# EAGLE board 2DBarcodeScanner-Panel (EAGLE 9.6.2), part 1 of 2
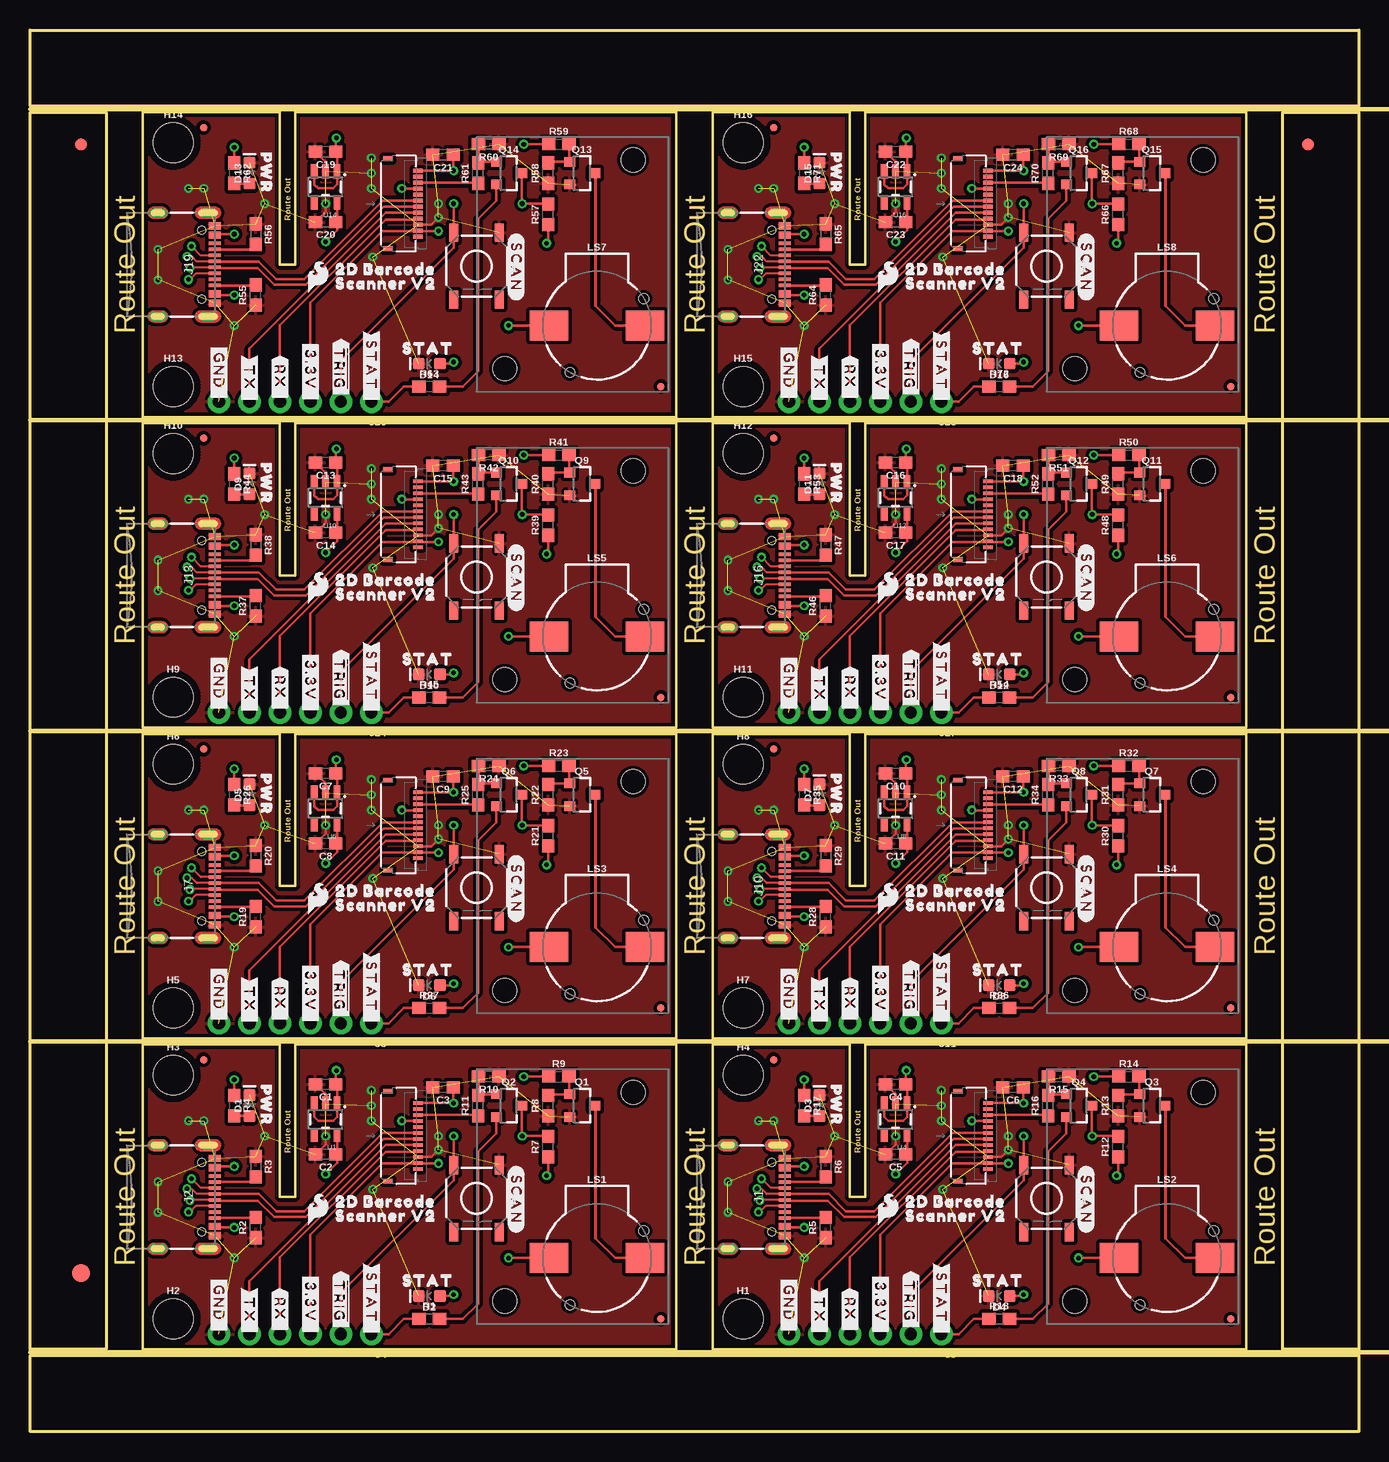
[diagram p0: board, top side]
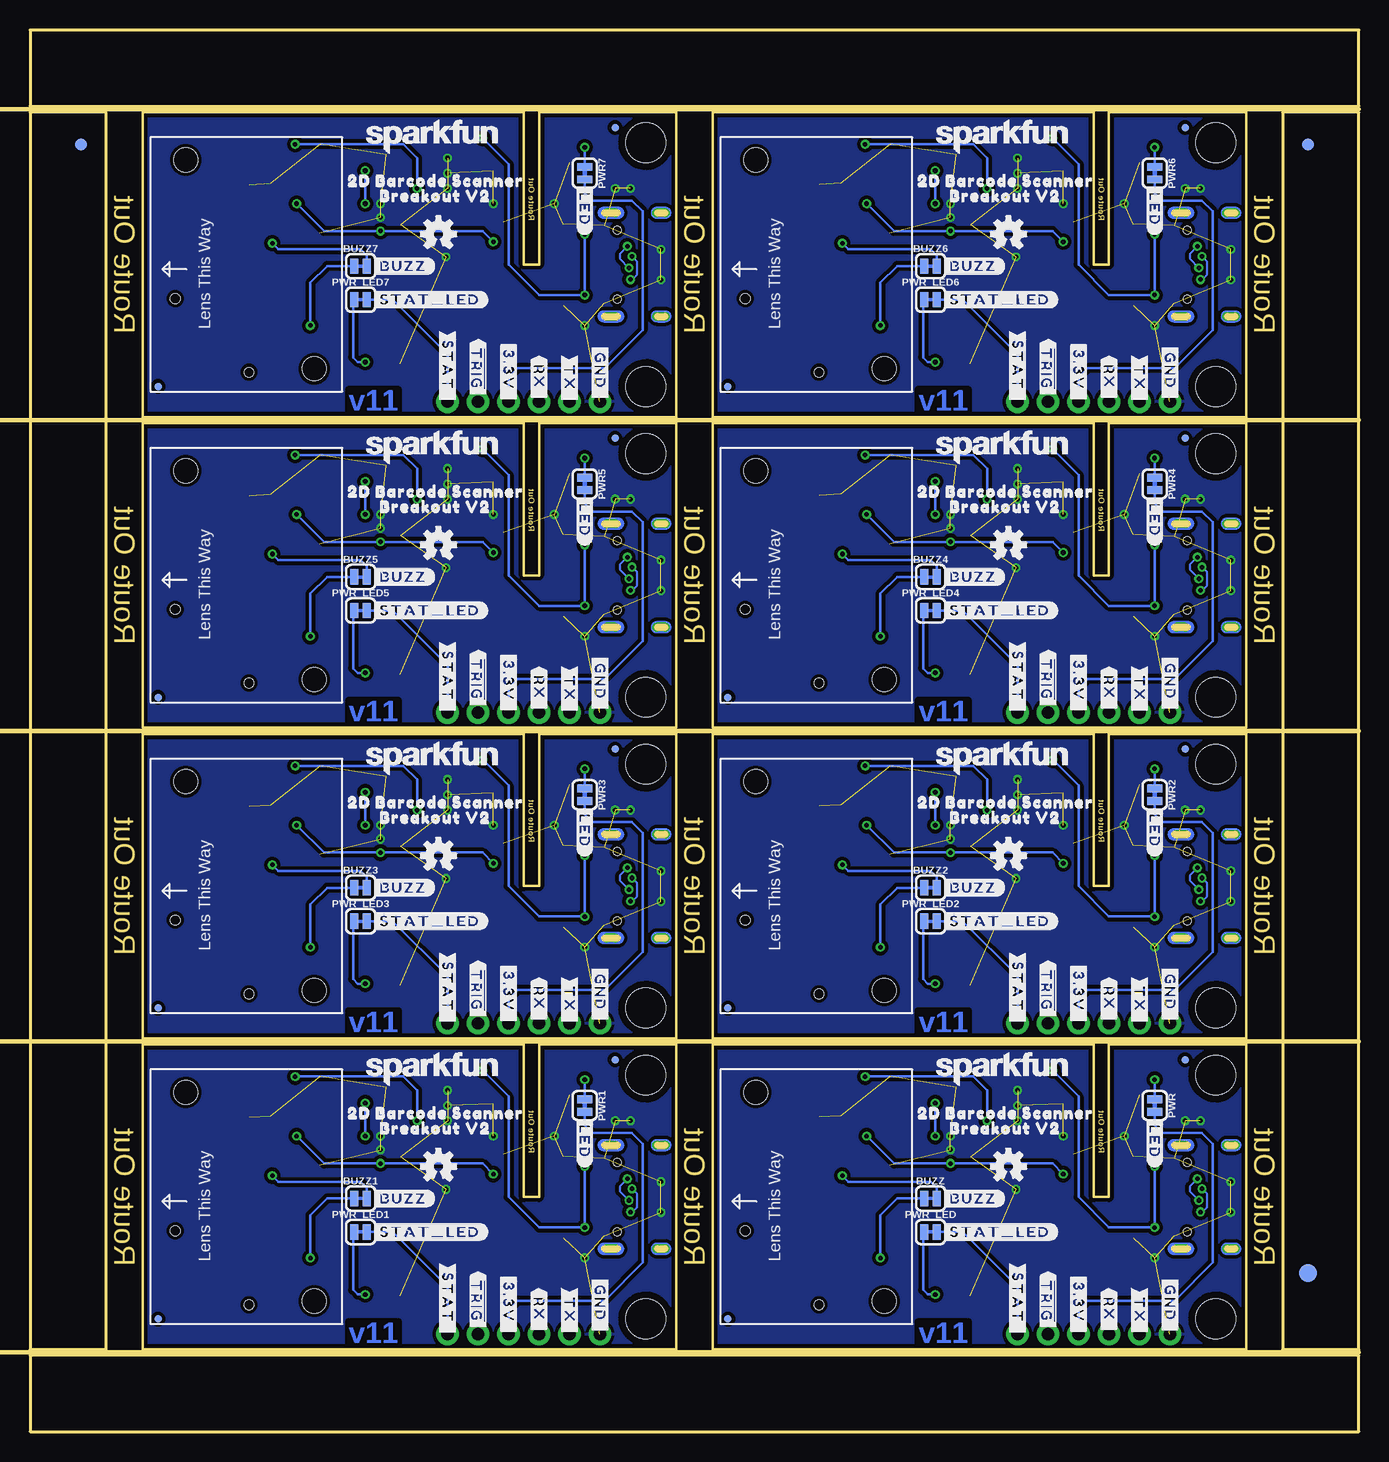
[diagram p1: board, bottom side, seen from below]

Size 110.74 x 116.84 mm. Coordinates in mm from the lower left corner, seen from the top.
Outline: 80 segments
Copper layers (1*16): Top 0.035mm / dielectric 1.5mm / Bottom 0.035mm
Design rules "2DBarcodeScanner": minimum track width 7mil, minimum drill 0.3mm, track to track 7mil, track to pad 7mil, pad to pad 7mil, via to via 7mil, smd to smd 7mil, copper to edge 7mil, drill to drill 7mil, minimum pad ring 7mil, minimum via ring 7mil, stop-mask expansion 3mil, vias tented up to drill 25mil, thermal gap 10mil
Net classes: 1 power: width 0.178 mm
Milling: 5 lines

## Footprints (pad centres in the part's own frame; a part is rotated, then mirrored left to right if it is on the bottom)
SMT-JUMPER_2_NC_TRACE_SILK = smd 0.66 x 1.27: 1 -0.521,0; 2 0.521,0
0603 = smd 1.1 x 1: 1 -0.85,0; 2 0.85,0
LED-0603 = smd 1 x 1: A -0.877,0; C 0.877,0
FIDUCIAL-1X2 = smd 1 x 1: 1 0,0
FIDUCIAL-1.5X3 = smd 1.5 x 1.5: 1 0,0
FIDUCIAL-MICRO = smd 0.635 x 0.635: 1 0,0
STAND-OFF = hole 3.302: 0,0
USB-C-16P-2LAYER-PADS = smd 0.3 x 1: A5 -1.25,-0.34; A6 -0.25,-0.34; A7 0.25,-0.34; A8 1.25,-0.34; B5 1.75,-0.34; B6 0.75,-0.34; B7 -0.75,-0.34; B8 -1.75,-0.34 | smd 0.6 x 1: GND -3.225,-0.34; GND2 3.225,-0.34; VBUS1 -2.45,-0.34; VBUS2 2.45,-0.34 | drill 0.4 pad 0.6 long: SHLD1 -4.318,-0.915; SHLD2 4.318,-0.915; SHLD3 -4.318,-5.095; SHLD4 4.318,-5.095 | hole 0.65: -2.89,-1.445; 2.89,-1.445
FPC_12_0.5MM = smd 0.3 x 0.8: 1 -2.75,1.35; 2 -2.25,1.35; 3 -1.75,1.35; 4 -1.25,1.35; 5 -0.75,1.35; 6 -0.25,1.35; 7 0.25,1.35; 8 0.75,1.35; 9 1.25,1.35; 10 1.75,1.35; 11 2.25,1.35; 12 2.75,1.35 | smd 0.4 x 0.8: MP1 -3.75,-1.15; MP2 3.75,-1.15
1X06_NO_SILK = drill 1.016 pad 1.88: 1 0,0; 2 2.54,0; 3 5.08,0; 4 7.62,0; 5 10.16,0; 6 12.7,0
BUZZER-CCV = smd 3.2 x 2.5: + 4,0; - -4,0 | hole 0.8: -3.9,-2.25; 2.25,3.9
SOT23-3 = smd 0.8 x 0.9: 1 -0.95,-1; 2 0.95,-1; 3 0,1.1
TACTILE_SWITCH_SMD_5.2MM = smd 1.524 x 0.762: 1 -2.794,1.905; 2 2.794,1.905; 3 -2.794,-1.905; 4 2.794,-1.905
SOT23-5 = smd 0.55 x 1.2: 1 -0.95,-1.3; 2 0,-1.3; 3 0.95,-1.3; 4 0.95,1.3; 5 -0.95,1.3
BARCODE_SCANNER_MOUNT = hole 2: -5.65,8.3; 5.05,-9.1

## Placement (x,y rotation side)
BUZZ  JUMPER-SMT_2_NC_TRACE_SILK  [SMT-JUMPER_2_NC_TRACE_SILK]  35.69,19.43 0 bottom
BUZZ1  JUMPER-SMT_2_NC_TRACE_SILK  [SMT-JUMPER_2_NC_TRACE_SILK]  83.19,19.43 0 bottom
BUZZ2  JUMPER-SMT_2_NC_TRACE_SILK  [SMT-JUMPER_2_NC_TRACE_SILK]  35.69,45.34 0 bottom
BUZZ3  JUMPER-SMT_2_NC_TRACE_SILK  [SMT-JUMPER_2_NC_TRACE_SILK]  83.19,45.34 0 bottom
BUZZ4  JUMPER-SMT_2_NC_TRACE_SILK  [SMT-JUMPER_2_NC_TRACE_SILK]  35.69,71.25 0 bottom
BUZZ5  JUMPER-SMT_2_NC_TRACE_SILK  [SMT-JUMPER_2_NC_TRACE_SILK]  83.19,71.25 0 bottom
BUZZ6  JUMPER-SMT_2_NC_TRACE_SILK  [SMT-JUMPER_2_NC_TRACE_SILK]  35.69,97.16 0 bottom
BUZZ7  JUMPER-SMT_2_NC_TRACE_SILK  [SMT-JUMPER_2_NC_TRACE_SILK]  83.19,97.16 0 bottom
C1  1.0uF  [0603]  24.64,28.96 180 top
C2  1.0uF  [0603]  24.64,23.11 180 top
C3  0.1uF  [0603]  34.42,28.7 180 top
C4  1.0uF  [0603]  72.14,28.96 180 top
C5  1.0uF  [0603]  72.14,23.11 180 top
C6  0.1uF  [0603]  81.91,28.7 180 top
C7  1.0uF  [0603]  24.64,54.86 180 top
C8  1.0uF  [0603]  24.64,49.02 180 top
C9  0.1uF  [0603]  34.42,54.61 180 top
C10  1.0uF  [0603]  72.14,54.86 180 top
C11  1.0uF  [0603]  72.14,49.02 180 top
C12  0.1uF  [0603]  81.91,54.61 180 top
C13  1.0uF  [0603]  24.64,80.77 180 top
C14  1.0uF  [0603]  24.64,74.93 180 top
C15  0.1uF  [0603]  34.42,80.52 180 top
C16  1.0uF  [0603]  72.14,80.77 180 top
C17  1.0uF  [0603]  72.14,74.93 180 top
C18  0.1uF  [0603]  81.91,80.52 180 top
C19  1.0uF  [0603]  24.64,106.68 180 top
C20  1.0uF  [0603]  24.64,100.84 180 top
C21  0.1uF  [0603]  34.42,106.43 180 top
C22  1.0uF  [0603]  72.14,106.68 180 top
C23  1.0uF  [0603]  72.14,100.84 180 top
C24  0.1uF  [0603]  81.91,106.43 180 top
D1  RED  [LED-0603]  18.29,27.18 90 top
D2  GREEN  [LED-0603]  33.27,11.3 180 top
D3  RED  [LED-0603]  65.79,27.18 90 top
D4  GREEN  [LED-0603]  80.77,11.3 180 top
D5  RED  [LED-0603]  18.29,53.09 90 top
D6  GREEN  [LED-0603]  33.27,37.21 180 top
D7  RED  [LED-0603]  65.79,53.09 90 top
D8  GREEN  [LED-0603]  80.77,37.21 180 top
D9  RED  [LED-0603]  18.29,78.99 90 top
D10  GREEN  [LED-0603]  33.27,63.12 180 top
D11  RED  [LED-0603]  65.79,78.99 90 top
D12  GREEN  [LED-0603]  80.77,63.12 180 top
D13  RED  [LED-0603]  18.29,104.9 90 top
D14  GREEN  [LED-0603]  33.27,89.03 180 top
D15  RED  [LED-0603]  65.79,104.9 90 top
D16  GREEN  [LED-0603]  80.77,89.03 180 top
E$1  [FIDUCIAL-1X2]  4.23,107.31 0 top
E$2  [FIDUCIAL-1X2]  4.23,107.31 0 bottom
E$3  [FIDUCIAL-1X2]  106.51,107.31 0 top
E$4  [FIDUCIAL-1X2]  106.51,107.31 0 bottom
E$5  [FIDUCIAL-1.5X3]  4.23,13.21 0 top
E$6  [FIDUCIAL-1.5X3]  4.23,13.21 0 bottom
FD1  FIDUCIALUFIDUCIAL  [FIDUCIAL-MICRO]  14.48,30.99 0 top
FD2  FIDUCIALUFIDUCIAL  [FIDUCIAL-MICRO]  52.58,9.4 0 top
FD3  FIDUCIALUFIDUCIAL  [FIDUCIAL-MICRO]  52.58,9.4 0 bottom
FD4  FIDUCIALUFIDUCIAL  [FIDUCIAL-MICRO]  14.48,30.99 0 bottom
FD5  FIDUCIALUFIDUCIAL  [FIDUCIAL-MICRO]  61.98,30.99 0 top
FD6  FIDUCIALUFIDUCIAL  [FIDUCIAL-MICRO]  100.08,9.4 0 top
FD7  FIDUCIALUFIDUCIAL  [FIDUCIAL-MICRO]  100.08,9.4 0 bottom
FD8  FIDUCIALUFIDUCIAL  [FIDUCIAL-MICRO]  61.98,30.99 0 bottom
FD9  FIDUCIALUFIDUCIAL  [FIDUCIAL-MICRO]  14.48,56.9 0 top
FD10  FIDUCIALUFIDUCIAL  [FIDUCIAL-MICRO]  52.58,35.31 0 top
FD11  FIDUCIALUFIDUCIAL  [FIDUCIAL-MICRO]  52.58,35.31 0 bottom
FD12  FIDUCIALUFIDUCIAL  [FIDUCIAL-MICRO]  14.48,56.9 0 bottom
FD13  FIDUCIALUFIDUCIAL  [FIDUCIAL-MICRO]  61.98,56.9 0 top
FD14  FIDUCIALUFIDUCIAL  [FIDUCIAL-MICRO]  100.08,35.31 0 top
FD15  FIDUCIALUFIDUCIAL  [FIDUCIAL-MICRO]  100.08,35.31 0 bottom
FD16  FIDUCIALUFIDUCIAL  [FIDUCIAL-MICRO]  61.98,56.9 0 bottom
FD17  FIDUCIALUFIDUCIAL  [FIDUCIAL-MICRO]  14.48,82.8 0 top
FD18  FIDUCIALUFIDUCIAL  [FIDUCIAL-MICRO]  52.58,61.21 0 top
FD19  FIDUCIALUFIDUCIAL  [FIDUCIAL-MICRO]  52.58,61.21 0 bottom
FD20  FIDUCIALUFIDUCIAL  [FIDUCIAL-MICRO]  14.48,82.8 0 bottom
FD21  FIDUCIALUFIDUCIAL  [FIDUCIAL-MICRO]  61.98,82.8 0 top
FD22  FIDUCIALUFIDUCIAL  [FIDUCIAL-MICRO]  100.08,61.21 0 top
FD23  FIDUCIALUFIDUCIAL  [FIDUCIAL-MICRO]  100.08,61.21 0 bottom
FD24  FIDUCIALUFIDUCIAL  [FIDUCIAL-MICRO]  61.98,82.8 0 bottom
FD25  FIDUCIALUFIDUCIAL  [FIDUCIAL-MICRO]  14.48,108.71 0 top
FD26  FIDUCIALUFIDUCIAL  [FIDUCIAL-MICRO]  52.58,87.12 0 top
FD27  FIDUCIALUFIDUCIAL  [FIDUCIAL-MICRO]  52.58,87.12 0 bottom
FD28  FIDUCIALUFIDUCIAL  [FIDUCIAL-MICRO]  14.48,108.71 0 bottom
FD29  FIDUCIALUFIDUCIAL  [FIDUCIAL-MICRO]  61.98,108.71 0 top
FD30  FIDUCIALUFIDUCIAL  [FIDUCIAL-MICRO]  100.08,87.12 0 top
FD31  FIDUCIALUFIDUCIAL  [FIDUCIAL-MICRO]  100.08,87.12 0 bottom
FD32  FIDUCIALUFIDUCIAL  [FIDUCIAL-MICRO]  61.98,108.71 0 bottom
H1  STAND-OFF  [STAND-OFF]  59.44,9.4 0 top
H2  STAND-OFF  [STAND-OFF]  11.94,9.4 0 top
H3  STAND-OFF  [STAND-OFF]  11.94,29.72 0 top
H4  STAND-OFF  [STAND-OFF]  59.44,29.72 0 top
H5  STAND-OFF  [STAND-OFF]  11.94,35.31 0 top
H6  STAND-OFF  [STAND-OFF]  11.94,55.63 0 top
H7  STAND-OFF  [STAND-OFF]  59.44,35.31 0 top
H8  STAND-OFF  [STAND-OFF]  59.44,55.63 0 top
H9  STAND-OFF  [STAND-OFF]  11.94,61.21 0 top
H10  STAND-OFF  [STAND-OFF]  11.94,81.53 0 top
H11  STAND-OFF  [STAND-OFF]  59.44,61.21 0 top
H12  STAND-OFF  [STAND-OFF]  59.44,81.53 0 top
H13  STAND-OFF  [STAND-OFF]  11.94,87.12 0 top
H14  STAND-OFF  [STAND-OFF]  11.94,107.44 0 top
H15  STAND-OFF  [STAND-OFF]  59.44,87.12 0 top
H16  STAND-OFF  [STAND-OFF]  59.44,107.44 0 top
J1  [USB-C-16P-2LAYER-PADS]  63.25,19.56 270 top
J2  [USB-C-16P-2LAYER-PADS]  15.75,19.56 270 top
J3  [FPC_12_0.5MM]  30.99,24.64 270 top
J4  [1X06_NO_SILK]  28.45,8.13 180 top
J5  [1X06_NO_SILK]  75.95,8.13 180 top
J6  [FPC_12_0.5MM]  78.49,24.64 270 top
J7  [USB-C-16P-2LAYER-PADS]  15.75,45.47 270 top
J8  [1X06_NO_SILK]  28.45,34.04 180 top
J9  [FPC_12_0.5MM]  30.99,50.55 270 top
J10  [USB-C-16P-2LAYER-PADS]  63.25,45.47 270 top
J11  [1X06_NO_SILK]  75.95,34.04 180 top
J12  [FPC_12_0.5MM]  78.49,50.55 270 top
J13  [USB-C-16P-2LAYER-PADS]  15.75,71.37 270 top
J14  [1X06_NO_SILK]  28.45,59.94 180 top
J15  [FPC_12_0.5MM]  30.99,76.45 270 top
J16  [USB-C-16P-2LAYER-PADS]  63.25,71.37 270 top
J17  [1X06_NO_SILK]  75.95,59.94 180 top
J18  [FPC_12_0.5MM]  78.49,76.45 270 top
J19  [USB-C-16P-2LAYER-PADS]  15.75,97.28 270 top
J20  [1X06_NO_SILK]  28.45,85.85 180 top
J21  [FPC_12_0.5MM]  30.99,102.36 270 top
J22  [USB-C-16P-2LAYER-PADS]  63.25,97.28 270 top
J23  [1X06_NO_SILK]  75.95,85.85 180 top
J24  [FPC_12_0.5MM]  78.49,102.36 270 top
LOGO1  OSHW-LOGOS  [OSHW-LOGO-S]  29.21,22.1 0 bottom
LOGO2  SFE_LOGO_FLAME.1_INCH  [SFE_LOGO_FLAME_.1]  24,18.54 0 top
LOGO3  SFE_LOGO_NAME.1_INCH  [SFE_LOGO_NAME_.1]  29.72,30.23 0 bottom
LOGO4  OSHW-LOGOS  [OSHW-LOGO-S]  76.71,22.1 0 bottom
LOGO5  SFE_LOGO_FLAME.1_INCH  [SFE_LOGO_FLAME_.1]  71.5,18.54 0 top
LOGO6  SFE_LOGO_NAME.1_INCH  [SFE_LOGO_NAME_.1]  77.22,30.23 0 bottom
LOGO7  OSHW-LOGOS  [OSHW-LOGO-S]  29.21,48.01 0 bottom
LOGO8  SFE_LOGO_FLAME.1_INCH  [SFE_LOGO_FLAME_.1]  24,44.45 0 top
LOGO9  SFE_LOGO_NAME.1_INCH  [SFE_LOGO_NAME_.1]  29.72,56.13 0 bottom
LOGO10  OSHW-LOGOS  [OSHW-LOGO-S]  76.71,48.01 0 bottom
LOGO11  SFE_LOGO_FLAME.1_INCH  [SFE_LOGO_FLAME_.1]  71.5,44.45 0 top
LOGO12  SFE_LOGO_NAME.1_INCH  [SFE_LOGO_NAME_.1]  77.22,56.13 0 bottom
LOGO13  OSHW-LOGOS  [OSHW-LOGO-S]  29.21,73.91 0 bottom
LOGO14  SFE_LOGO_FLAME.1_INCH  [SFE_LOGO_FLAME_.1]  24,70.36 0 top
LOGO15  SFE_LOGO_NAME.1_INCH  [SFE_LOGO_NAME_.1]  29.72,82.04 0 bottom
LOGO16  OSHW-LOGOS  [OSHW-LOGO-S]  76.71,73.91 0 bottom
LOGO17  SFE_LOGO_FLAME.1_INCH  [SFE_LOGO_FLAME_.1]  71.5,70.36 0 top
LOGO18  SFE_LOGO_NAME.1_INCH  [SFE_LOGO_NAME_.1]  77.22,82.04 0 bottom
LOGO19  OSHW-LOGOS  [OSHW-LOGO-S]  29.21,99.82 0 bottom
LOGO20  SFE_LOGO_FLAME.1_INCH  [SFE_LOGO_FLAME_.1]  24,96.27 0 top
LOGO21  SFE_LOGO_NAME.1_INCH  [SFE_LOGO_NAME_.1]  29.72,107.95 0 bottom
LOGO22  OSHW-LOGOS  [OSHW-LOGO-S]  76.71,99.82 0 bottom
LOGO23  SFE_LOGO_FLAME.1_INCH  [SFE_LOGO_FLAME_.1]  71.5,96.27 0 top
LOGO24  SFE_LOGO_NAME.1_INCH  [SFE_LOGO_NAME_.1]  77.22,107.95 0 bottom
LS1  BUZZER-SMD  [BUZZER-CCV]  47.24,14.48 180 top
LS2  BUZZER-SMD  [BUZZER-CCV]  94.74,14.48 180 top
LS3  BUZZER-SMD  [BUZZER-CCV]  47.24,40.39 180 top
LS4  BUZZER-SMD  [BUZZER-CCV]  94.74,40.39 180 top
LS5  BUZZER-SMD  [BUZZER-CCV]  47.24,66.29 180 top
LS6  BUZZER-SMD  [BUZZER-CCV]  94.74,66.29 180 top
LS7  BUZZER-SMD  [BUZZER-CCV]  47.24,92.2 180 top
LS8  BUZZER-SMD  [BUZZER-CCV]  94.74,92.2 180 top
PWR  JUMPER-SMT_2_NC_TRACE_SILK  [SMT-JUMPER_2_NC_TRACE_SILK]  17.02,27.18 270 bottom
PWR1  JUMPER-SMT_2_NC_TRACE_SILK  [SMT-JUMPER_2_NC_TRACE_SILK]  64.52,27.18 270 bottom
PWR2  JUMPER-SMT_2_NC_TRACE_SILK  [SMT-JUMPER_2_NC_TRACE_SILK]  17.02,53.09 270 bottom
PWR3  JUMPER-SMT_2_NC_TRACE_SILK  [SMT-JUMPER_2_NC_TRACE_SILK]  64.52,53.09 270 bottom
PWR4  JUMPER-SMT_2_NC_TRACE_SILK  [SMT-JUMPER_2_NC_TRACE_SILK]  17.02,78.99 270 bottom
PWR5  JUMPER-SMT_2_NC_TRACE_SILK  [SMT-JUMPER_2_NC_TRACE_SILK]  64.52,78.99 270 bottom
PWR6  JUMPER-SMT_2_NC_TRACE_SILK  [SMT-JUMPER_2_NC_TRACE_SILK]  17.02,104.9 270 bottom
PWR7  JUMPER-SMT_2_NC_TRACE_SILK  [SMT-JUMPER_2_NC_TRACE_SILK]  64.52,104.9 270 bottom
PWR_LED  JUMPER-SMT_2_NC_TRACE_SILK  [SMT-JUMPER_2_NC_TRACE_SILK]  35.69,16.64 0 bottom
PWR_LED1  JUMPER-SMT_2_NC_TRACE_SILK  [SMT-JUMPER_2_NC_TRACE_SILK]  83.19,16.64 0 bottom
PWR_LED2  JUMPER-SMT_2_NC_TRACE_SILK  [SMT-JUMPER_2_NC_TRACE_SILK]  35.69,42.54 0 bottom
PWR_LED3  JUMPER-SMT_2_NC_TRACE_SILK  [SMT-JUMPER_2_NC_TRACE_SILK]  83.19,42.54 0 bottom
PWR_LED4  JUMPER-SMT_2_NC_TRACE_SILK  [SMT-JUMPER_2_NC_TRACE_SILK]  35.69,68.45 0 bottom
PWR_LED5  JUMPER-SMT_2_NC_TRACE_SILK  [SMT-JUMPER_2_NC_TRACE_SILK]  83.19,68.45 0 bottom
PWR_LED6  JUMPER-SMT_2_NC_TRACE_SILK  [SMT-JUMPER_2_NC_TRACE_SILK]  35.69,94.36 0 bottom
PWR_LED7  JUMPER-SMT_2_NC_TRACE_SILK  [SMT-JUMPER_2_NC_TRACE_SILK]  83.19,94.36 0 bottom
Q1  600mA/40V  [SOT23-3]  45.97,27.18 270 top
Q2  600mA/40V  [SOT23-3]  39.88,27.18 270 top
Q3  600mA/40V  [SOT23-3]  93.47,27.18 270 top
Q4  600mA/40V  [SOT23-3]  87.38,27.18 270 top
Q5  600mA/40V  [SOT23-3]  45.97,53.09 270 top
Q6  600mA/40V  [SOT23-3]  39.88,53.09 270 top
Q7  600mA/40V  [SOT23-3]  93.47,53.09 270 top
Q8  600mA/40V  [SOT23-3]  87.38,53.09 270 top
Q9  600mA/40V  [SOT23-3]  45.97,78.99 270 top
Q10  600mA/40V  [SOT23-3]  39.88,78.99 270 top
Q11  600mA/40V  [SOT23-3]  93.47,78.99 270 top
Q12  600mA/40V  [SOT23-3]  87.38,78.99 270 top
Q13  600mA/40V  [SOT23-3]  45.97,104.9 270 top
Q14  600mA/40V  [SOT23-3]  39.88,104.9 270 top
Q15  600mA/40V  [SOT23-3]  93.47,104.9 270 top
Q16  600mA/40V  [SOT23-3]  87.38,104.9 270 top
R1  100  [0603]  33.27,9.4 0 top
R2  5.1k  [0603]  18.8,17.02 90 top
R3  5.1k  [0603]  18.8,22.1 270 top
R4  1k  [0603]  17.02,27.18 270 top
R5  5.1k  [0603]  66.29,17.02 90 top
R6  5.1k  [0603]  66.29,22.1 270 top
R7  10  [0603]  43.18,23.75 90 top
R8  10k  [0603]  43.18,27.18 90 top
R9  1k  [0603]  44.07,29.59 0 top
R10  10k  [0603]  38.23,29.59 180 top
R11  1k  [0603]  37.34,27.18 90 top
R12  10  [0603]  90.68,23.75 90 top
R13  10k  [0603]  90.68,27.18 90 top
R14  1k  [0603]  91.57,29.59 0 top
R15  10k  [0603]  85.72,29.59 180 top
R16  1k  [0603]  84.84,27.18 90 top
R17  1k  [0603]  64.52,27.18 270 top
R18  100  [0603]  80.77,9.4 0 top
R19  5.1k  [0603]  18.8,42.93 90 top
R20  5.1k  [0603]  18.8,48.01 270 top
R21  10  [0603]  43.18,49.66 90 top
R22  10k  [0603]  43.18,53.09 90 top
R23  1k  [0603]  44.07,55.5 0 top
R24  10k  [0603]  38.23,55.5 180 top
R25  1k  [0603]  37.34,53.09 90 top
R26  1k  [0603]  17.02,53.09 270 top
R27  100  [0603]  33.27,35.31 0 top
R28  5.1k  [0603]  66.29,42.93 90 top
R29  5.1k  [0603]  66.29,48.01 270 top
R30  10  [0603]  90.68,49.66 90 top
R31  10k  [0603]  90.68,53.09 90 top
R32  1k  [0603]  91.57,55.5 0 top
R33  10k  [0603]  85.72,55.5 180 top
R34  1k  [0603]  84.84,53.09 90 top
R35  1k  [0603]  64.52,53.09 270 top
R36  100  [0603]  80.77,35.31 0 top
R37  5.1k  [0603]  18.8,68.83 90 top
R38  5.1k  [0603]  18.8,73.91 270 top
R39  10  [0603]  43.18,75.56 90 top
R40  10k  [0603]  43.18,78.99 90 top
R41  1k  [0603]  44.07,81.41 0 top
R42  10k  [0603]  38.23,81.41 180 top
R43  1k  [0603]  37.34,78.99 90 top
R44  1k  [0603]  17.02,78.99 270 top
R45  100  [0603]  33.27,61.21 0 top
R46  5.1k  [0603]  66.29,68.83 90 top
R47  5.1k  [0603]  66.29,73.91 270 top
R48  10  [0603]  90.68,75.56 90 top
R49  10k  [0603]  90.68,78.99 90 top
R50  1k  [0603]  91.57,81.41 0 top
R51  10k  [0603]  85.72,81.41 180 top
R52  1k  [0603]  84.84,78.99 90 top
R53  1k  [0603]  64.52,78.99 270 top
R54  100  [0603]  80.77,61.21 0 top
R55  5.1k  [0603]  18.8,94.74 90 top
R56  5.1k  [0603]  18.8,99.82 270 top
R57  10  [0603]  43.18,101.47 90 top
R58  10k  [0603]  43.18,104.9 90 top
R59  1k  [0603]  44.07,107.31 0 top
R60  10k  [0603]  38.23,107.31 180 top
R61  1k  [0603]  37.34,104.9 90 top
R62  1k  [0603]  17.02,104.9 270 top
R63  100  [0603]  33.27,87.12 0 top
R64  5.1k  [0603]  66.29,94.74 90 top
R65  5.1k  [0603]  66.29,99.82 270 top
R66  10  [0603]  90.68,101.47 90 top
R67  10k  [0603]  90.68,104.9 90 top
R68  1k  [0603]  91.57,107.31 0 top
R69  10k  [0603]  85.72,107.31 180 top
R70  1k  [0603]  84.84,104.9 90 top
R71  1k  [0603]  64.52,104.9 270 top
R72  100  [0603]  80.77,87.12 0 top
S1  MOMENTARY-SWITCH-SPST-SMD-5.2MM-TALL  [TACTILE_SWITCH_SMD_5.2MM]  84.71,19.43 270 top
S2  MOMENTARY-SWITCH-SPST-SMD-5.2MM-TALL  [TACTILE_SWITCH_SMD_5.2MM]  37.21,19.43 270 top
S3  MOMENTARY-SWITCH-SPST-SMD-5.2MM-TALL  [TACTILE_SWITCH_SMD_5.2MM]  37.21,45.34 270 top
S4  MOMENTARY-SWITCH-SPST-SMD-5.2MM-TALL  [TACTILE_SWITCH_SMD_5.2MM]  84.71,45.34 270 top
S5  MOMENTARY-SWITCH-SPST-SMD-5.2MM-TALL  [TACTILE_SWITCH_SMD_5.2MM]  37.21,71.25 270 top
S6  MOMENTARY-SWITCH-SPST-SMD-5.2MM-TALL  [TACTILE_SWITCH_SMD_5.2MM]  84.71,71.25 270 top
S7  MOMENTARY-SWITCH-SPST-SMD-5.2MM-TALL  [TACTILE_SWITCH_SMD_5.2MM]  37.21,97.16 270 top
S8  MOMENTARY-SWITCH-SPST-SMD-5.2MM-TALL  [TACTILE_SWITCH_SMD_5.2MM]  84.71,97.16 270 top
U1  3.3V  [SOT23-5]  24.64,26.04 180 top
U2  BARCODE_SCANNER_MOUNT  [BARCODE_SCANNER_MOUNT]  45.21,19.18 180 bottom
U3  BARCODE_SCANNER_MOUNT  [BARCODE_SCANNER_MOUNT]  92.71,19.18 180 bottom
U4  3.3V  [SOT23-5]  72.14,26.04 180 top
U5  BARCODE_SCANNER_MOUNT  [BARCODE_SCANNER_MOUNT]  45.21,45.08 180 bottom
U6  3.3V  [SOT23-5]  24.64,51.94 180 top
U7  BARCODE_SCANNER_MOUNT  [BARCODE_SCANNER_MOUNT]  92.71,45.08 180 bottom
U8  3.3V  [SOT23-5]  72.14,51.94 180 top
U9  BARCODE_SCANNER_MOUNT  [BARCODE_SCANNER_MOUNT]  45.21,70.99 180 bottom
U10  3.3V  [SOT23-5]  24.64,77.85 180 top
U11  BARCODE_SCANNER_MOUNT  [BARCODE_SCANNER_MOUNT]  92.71,70.99 180 bottom
U12  3.3V  [SOT23-5]  72.14,77.85 180 top
U13  BARCODE_SCANNER_MOUNT  [BARCODE_SCANNER_MOUNT]  45.21,96.9 180 bottom
U14  3.3V  [SOT23-5]  24.64,103.76 180 top
U15  BARCODE_SCANNER_MOUNT  [BARCODE_SCANNER_MOUNT]  92.71,96.9 180 bottom
U16  3.3V  [SOT23-5]  72.14,103.76 180 top
U$1  [##TRIG##0]  25.91,13.34 270 top
U$2  [#STAT_#0]  28.45,13.97 270 top
U$3  [STAT0]  30.35,12.57 0 top
U$4  [#SCAN#0]  40.51,22.1 270 top
U$5  [#BUZZ#0]  34.8,19.43 0 bottom
U$6  [#STAT_LED#0]  34.8,16.64 0 bottom
U$7  [##TRIG##0]  25.91,13.34 270 bottom
U$8  [PWR0]  19.69,29.59 270 top
U$9  [#LED#0]  17.02,26.29 270 bottom
U$10  [SCANNER_V20]  24.77,17.98 0 top
U$11  [BREAKOUT_V20]  34.8,25.27 0 bottom
U$12  [2D_BARCODE_SCANNER0]  37.47,26.54 0 bottom
U$13  [#STAT_#0]  75.95,13.97 270 top
U$14  [STAT0]  77.85,12.57 0 top
U$15  [2D_BARCODE0]  72.26,19.18 0 top
U$16  [#STAT_#0]  75.95,13.97 270 bottom
U$17  [2D_BARCODE0]  24.77,19.18 0 top
U$18  [#3#3V_#0]  70.87,13.21 270 top
U$19  [#3#3V_#0]  70.87,13.21 270 bottom
U$20  [#TX_#0]  65.79,11.94 270 top
U$21  [#STAT_#0]  28.45,13.97 270 bottom
U$22  [#TX_#0]  65.79,11.94 270 bottom
U$23  [#RX_#0]  68.33,11.94 270 top
U$24  [#RX_#0]  68.33,11.94 270 bottom
U$25  [#GND_#0]  63.25,12.95 270 top
U$26  [#TX_#0]  18.29,11.94 270 top
U$27  [#TX_#0]  18.29,11.94 270 bottom
U$28  [#3#3V_#0]  23.37,13.21 270 top
U$29  [#3#3V_#0]  23.37,13.21 270 bottom
U$30  [#RX_#0]  20.83,11.94 270 top
U$31  [#RX_#0]  20.83,11.94 270 bottom
U$32  [#GND_#0]  15.75,12.95 270 top
U$33  [#GND_#0]  15.75,12.95 270 bottom
U$34  [#GND_#0]  63.25,12.95 270 bottom
U$35  [#SCAN#0]  88.01,22.1 270 top
U$36  [#BUZZ#0]  82.3,19.43 0 bottom
U$37  [PWR0]  67.18,29.59 270 top
U$38  [#LED#0]  64.52,26.29 270 bottom
U$39  [#STAT_LED#0]  82.3,16.64 0 bottom
U$40  [##TRIG##0]  73.41,13.34 270 top
U$41  [##TRIG##0]  73.41,13.34 270 bottom
U$42  [SCANNER_V20]  72.26,17.98 0 top
U$43  [BREAKOUT_V20]  82.3,25.27 0 bottom
U$44  [2D_BARCODE_SCANNER0]  84.96,26.54 0 bottom
U$45  [#STAT_#0]  28.45,39.88 270 top
U$46  [STAT0]  30.35,38.48 0 top
U$47  [2D_BARCODE0]  24.77,45.08 0 top
U$48  [#STAT_#0]  28.45,39.88 270 bottom
U$49  [#3#3V_#0]  23.37,39.12 270 top
U$50  [#3#3V_#0]  23.37,39.12 270 bottom
U$51  [#TX_#0]  18.29,37.85 270 top
U$52  [#TX_#0]  18.29,37.85 270 bottom
U$53  [#RX_#0]  20.83,37.85 270 top
U$54  [#RX_#0]  20.83,37.85 270 bottom
U$55  [#GND_#0]  15.75,38.86 270 top
U$56  [#GND_#0]  15.75,38.86 270 bottom
U$57  [#SCAN#0]  40.51,48.01 270 top
U$58  [#BUZZ#0]  34.8,45.34 0 bottom
U$59  [PWR0]  19.69,55.5 270 top
U$60  [#LED#0]  17.02,52.2 270 bottom
U$61  [#STAT_LED#0]  34.8,42.54 0 bottom
U$62  [##TRIG##0]  25.91,39.24 270 top
U$63  [##TRIG##0]  25.91,39.24 270 bottom
U$64  [SCANNER_V20]  24.77,43.89 0 top
U$65  [BREAKOUT_V20]  34.8,51.18 0 bottom
U$66  [2D_BARCODE_SCANNER0]  37.47,52.45 0 bottom
U$67  [#STAT_#0]  75.95,39.88 270 top
U$68  [STAT0]  77.85,38.48 0 top
U$69  [2D_BARCODE0]  72.26,45.08 0 top
U$70  [#STAT_#0]  75.95,39.88 270 bottom
U$71  [#3#3V_#0]  70.87,39.12 270 top
U$72  [#3#3V_#0]  70.87,39.12 270 bottom
U$73  [#TX_#0]  65.79,37.85 270 top
U$74  [#TX_#0]  65.79,37.85 270 bottom
U$75  [#RX_#0]  68.33,37.85 270 top
U$76  [#RX_#0]  68.33,37.85 270 bottom
U$77  [#GND_#0]  63.25,38.86 270 top
U$78  [#GND_#0]  63.25,38.86 270 bottom
U$79  [#SCAN#0]  88.01,48.01 270 top
U$80  [#BUZZ#0]  82.3,45.34 0 bottom
U$81  [PWR0]  67.18,55.5 270 top
U$82  [#LED#0]  64.52,52.2 270 bottom
U$83  [#STAT_LED#0]  82.3,42.54 0 bottom
U$84  [##TRIG##0]  73.41,39.24 270 top
U$85  [##TRIG##0]  73.41,39.24 270 bottom
U$86  [SCANNER_V20]  72.26,43.89 0 top
U$87  [BREAKOUT_V20]  82.3,51.18 0 bottom
U$88  [2D_BARCODE_SCANNER0]  84.96,52.45 0 bottom
U$89  [#STAT_#0]  28.45,65.79 270 top
U$90  [STAT0]  30.35,64.39 0 top
U$91  [2D_BARCODE0]  24.77,70.99 0 top
U$92  [#STAT_#0]  28.45,65.79 270 bottom
U$93  [#3#3V_#0]  23.37,65.02 270 top
U$94  [#3#3V_#0]  23.37,65.02 270 bottom
U$95  [#TX_#0]  18.29,63.75 270 top
U$96  [#TX_#0]  18.29,63.75 270 bottom
U$97  [#RX_#0]  20.83,63.75 270 top
U$98  [#RX_#0]  20.83,63.75 270 bottom
U$99  [#GND_#0]  15.75,64.77 270 top
U$100  [#GND_#0]  15.75,64.77 270 bottom
U$101  [#SCAN#0]  40.51,73.91 270 top
U$102  [#BUZZ#0]  34.8,71.25 0 bottom
U$103  [PWR0]  19.69,81.41 270 top
U$104  [#LED#0]  17.02,78.11 270 bottom
U$105  [#STAT_LED#0]  34.8,68.45 0 bottom
U$106  [##TRIG##0]  25.91,65.15 270 top
U$107  [##TRIG##0]  25.91,65.15 270 bottom
U$108  [SCANNER_V20]  24.77,69.8 0 top
U$109  [BREAKOUT_V20]  34.8,77.09 0 bottom
U$110  [2D_BARCODE_SCANNER0]  37.47,78.36 0 bottom
U$111  [#STAT_#0]  75.95,65.79 270 top
U$112  [STAT0]  77.85,64.39 0 top
U$113  [2D_BARCODE0]  72.26,70.99 0 top
U$114  [#STAT_#0]  75.95,65.79 270 bottom
U$115  [#3#3V_#0]  70.87,65.02 270 top
U$116  [#3#3V_#0]  70.87,65.02 270 bottom
U$117  [#TX_#0]  65.79,63.75 270 top
U$118  [#TX_#0]  65.79,63.75 270 bottom
U$119  [#RX_#0]  68.33,63.75 270 top
U$120  [#RX_#0]  68.33,63.75 270 bottom
U$121  [#GND_#0]  63.25,64.77 270 top
U$122  [#GND_#0]  63.25,64.77 270 bottom
U$123  [#SCAN#0]  88.01,73.91 270 top
U$124  [#BUZZ#0]  82.3,71.25 0 bottom
U$125  [PWR0]  67.18,81.41 270 top
U$126  [#LED#0]  64.52,78.11 270 bottom
U$127  [#STAT_LED#0]  82.3,68.45 0 bottom
U$128  [##TRIG##0]  73.41,65.15 270 top
U$129  [##TRIG##0]  73.41,65.15 270 bottom
U$130  [SCANNER_V20]  72.26,69.8 0 top
U$131  [BREAKOUT_V20]  82.3,77.09 0 bottom
U$132  [2D_BARCODE_SCANNER0]  84.96,78.36 0 bottom
U$133  [#STAT_#0]  28.45,91.69 270 top
U$134  [STAT0]  30.35,90.3 0 top
U$135  [2D_BARCODE0]  24.77,96.9 0 top
U$136  [#STAT_#0]  28.45,91.69 270 bottom
U$137  [#3#3V_#0]  23.37,90.93 270 top
U$138  [#3#3V_#0]  23.37,90.93 270 bottom
U$139  [#TX_#0]  18.29,89.66 270 top
U$140  [#TX_#0]  18.29,89.66 270 bottom
U$141  [#RX_#0]  20.83,89.66 270 top
U$142  [#RX_#0]  20.83,89.66 270 bottom
U$143  [#GND_#0]  15.75,90.68 270 top
U$144  [#GND_#0]  15.75,90.68 270 bottom
U$145  [#SCAN#0]  40.51,99.82 270 top
U$146  [#BUZZ#0]  34.8,97.16 0 bottom
U$147  [PWR0]  19.69,107.31 270 top
U$148  [#LED#0]  17.02,104.01 270 bottom
U$149  [#STAT_LED#0]  34.8,94.36 0 bottom
U$150  [##TRIG##0]  25.91,91.06 270 top
U$151  [##TRIG##0]  25.91,91.06 270 bottom
U$152  [SCANNER_V20]  24.77,95.71 0 top
U$153  [BREAKOUT_V20]  34.8,103 0 bottom
U$154  [2D_BARCODE_SCANNER0]  37.47,104.27 0 bottom
U$155  [#STAT_#0]  75.95,91.69 270 top
U$156  [STAT0]  77.85,90.3 0 top
U$157  [2D_BARCODE0]  72.26,96.9 0 top
U$158  [#STAT_#0]  75.95,91.69 270 bottom
U$159  [#3#3V_#0]  70.87,90.93 270 top
U$160  [#3#3V_#0]  70.87,90.93 270 bottom
U$161  [#TX_#0]  65.79,89.66 270 top
U$162  [#TX_#0]  65.79,89.66 270 bottom
U$163  [#RX_#0]  68.33,89.66 270 top
U$164  [#RX_#0]  68.33,89.66 270 bottom
U$165  [#GND_#0]  63.25,90.68 270 top
U$166  [#GND_#0]  63.25,90.68 270 bottom
U$167  [#SCAN#0]  88.01,99.82 270 top
U$168  [#BUZZ#0]  82.3,97.16 0 bottom
U$169  [PWR0]  67.18,107.31 270 top
U$170  [#LED#0]  64.52,104.01 270 bottom
U$171  [#STAT_LED#0]  82.3,94.36 0 bottom
U$172  [##TRIG##0]  73.41,91.06 270 top
U$173  [##TRIG##0]  73.41,91.06 270 bottom
U$174  [SCANNER_V20]  72.26,95.71 0 top
U$175  [BREAKOUT_V20]  82.3,103 0 bottom
U$176  [2D_BARCODE_SCANNER0]  84.96,104.27 0 bottom

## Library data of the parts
BUZZ BUZZ1-BUZZ7 PWR PWR1-PWR7 PWR_LED PWR_LED1-PWR_LED7 = SparkFun-Jumpers
C1 C2 C4 C5 C7 C8 C10 C11 C13 C14 C16 C17 C19 C20 C22 C23 = SparkFun-Capacitors; PROD_ID: CAP-00868
C3 C6 C9 C12 C15 C18 C21 C24 = SparkFun-Capacitors; PROD_ID: CAP-00810
D1 D3 D5 D7 D9 D11 D13 D15 = SparkFun-LED; PROD_ID: DIO-00819
D2 D4 D6 D8 D10 D12 D14 D16 = SparkFun-LED; PROD_ID: DIO-00821
E$1-E$4 FD1-FD32 LOGO1-LOGO24 = SparkFun-Aesthetics
E$5 E$6 = SparkFun-Retired
H1-H16 = SparkFun-Hardware
J1 J2 J7 J10 J13 J16 J19 J22 = SparkFun-Connectors; PROD_ID: CONN-14122
J3 J6 J9 J12 J15 J18 J21 J24 = SparkFun-Connectors; PROD_ID: CONN-15766
J4 J5 J8 J11 J14 J17 J20 J23 = SparkFun-Connectors; PROD_ID: CONN-08437
LS1-LS8 = SparkFun-Electromechanical; PROD_ID: COMP-08568
Q1-Q16 = SparkFun-DiscreteSemi; PROD_ID: TRANS-08049
R1 R18 R27 R36 R45 R54 R63 R72 = SparkFun-Resistors; PROD_ID: RES-07863
R2 R3 R5 R6 R19 R20 R28 R29 R37 R38 R46 R47 R55 R56 R64 R65 = SparkFun-Resistors; PROD_ID: RES-12083
R4 R9 R11 R14 R16 R17 R23 R25 R26 R32 R34 R35 R41 R43 R44 R50 R52 R53 R59 R61 R62 R68 R70 R71 = SparkFun-Resistors; PROD_ID: RES-07856
R7 R12 R21 R30 R39 R48 R57 R66 = SparkFun-Resistors; PROD_ID: RES-09834
R8 R10 R13 R15 R22 R24 R31 R33 R40 R42 R49 R51 R58 R60 R67 R69 = SparkFun-Resistors; PROD_ID: RES-00824
S1-S8 = SparkFun-Switches; PROD_ID: SWCH-14139
U1 U4 U6 U8 U10 U12 U14 U16 = SparkFun-IC-Power; PROD_ID: VREG-12457
U2 U3 U5 U7 U9 U11 U13 U15 = SparkFun-Hardware; PROD_ID: LPA-14926
U$1-U$9 U$13-U$41 U$45-U$63 U$67-U$85 U$89-U$107 U$111-U$129 U$133-U$151 U$155-U$173 = output
U$10 U$42 U$64 U$86 U$108 U$130 U$152 U$174 = SCANNER_V2
U$11 U$43 U$65 U$87 U$109 U$131 U$153 U$175 = BREAKOUT_V2
U$12 U$44 U$66 U$88 U$110 U$132 U$154 U$176 = 2D_BARCODE_SCANNER

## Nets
3.3V [power]: C2.1 J3.11 J4.3 PWR.2 Q2.3 R7.2 U1.5
3.3V1 [power]: C5.1 J5.3 J6.11 PWR1.2 Q4.3 R12.2 U4.5
3.3V2 [power]: C8.1 J8.3 J9.11 PWR2.2 Q6.3 R21.2 U6.5
3.3V3 [power]: C11.1 J11.3 J12.11 PWR3.2 Q8.3 R30.2 U8.5
3.3V4 [power]: C14.1 J14.3 J15.11 PWR4.2 Q10.3 R39.2 U10.5
3.3V5 [power]: C17.1 J17.3 J18.11 PWR5.2 Q12.3 R48.2 U12.5
3.3V6 [power]: C20.1 J20.3 J21.11 PWR6.2 Q14.3 R57.2 U14.5
3.3V7 [power]: C23.1 J23.3 J24.11 PWR7.2 Q16.3 R66.2 U16.5
5V: C1.1 J2.VBUS1 J2.VBUS2 U1.1 U1.3
5V1: C4.1 J1.VBUS1 J1.VBUS2 U4.1 U4.3
5V2: C7.1 J7.VBUS1 J7.VBUS2 U6.1 U6.3
5V3: C10.1 J10.VBUS1 J10.VBUS2 U8.1 U8.3
5V4: C13.1 J13.VBUS1 J13.VBUS2 U10.1 U10.3
5V5: C16.1 J16.VBUS1 J16.VBUS2 U12.1 U12.3
5V6: C19.1 J19.VBUS1 J19.VBUS2 U14.1 U14.3
5V7: C22.1 J22.VBUS1 J22.VBUS2 U16.1 U16.3
!SCAN_TRIGGER!: C3.1 J3.1 J4.2 S2.3
!SCAN_TRIGGER!1: C6.1 J5.2 J6.1 S1.3
!SCAN_TRIGGER!2: C9.1 J8.2 J9.1 S3.3
!SCAN_TRIGGER!3: C12.1 J11.2 J12.1 S4.3
!SCAN_TRIGGER!4: C15.1 J14.2 J15.1 S5.3
!SCAN_TRIGGER!5: C18.1 J17.2 J18.1 S6.3
!SCAN_TRIGGER!6: C21.1 J20.2 J21.1 S7.3
!SCAN_TRIGGER!7: C24.1 J23.2 J24.1 S8.3
BUZZER: J3.4 R9.1
BUZZER1: J6.4 R14.1
BUZZER2: J9.4 R23.1
BUZZER3: J12.4 R32.1
BUZZER4: J15.4 R41.1
BUZZER5: J18.4 R50.1
BUZZER6: J21.4 R59.1
BUZZER7: J24.4 R68.1
CC1: J1.A5 R6.2
CC2: J1.B5 R5.2
CC3: J2.A5 R3.2
CC4: J2.B5 R2.2
CC5: J7.A5 R20.2
CC6: J7.B5 R19.2
CC7: J10.A5 R29.2
CC8: J10.B5 R28.2
CC9: J13.A5 R38.2
CC10: J13.B5 R37.2
CC11: J16.A5 R47.2
CC12: J16.B5 R46.2
CC13: J19.A5 R56.2
CC14: J19.B5 R55.2
CC15: J22.A5 R65.2
CC16: J22.B5 R64.2
GND [power]: C1.2 C2.2 C3.2 D1.C D2.C J2.GND J2.GND2 J3.10 J4.6 Q1.2 R2.1 R3.1 R8.1 R10.1 S2.1 U1.2
GND1 [power]: C4.2 C5.2 C6.2 D3.C D4.C J1.GND J1.GND2 J5.6 J6.10 Q3.2 R5.1 R6.1 R13.1 R15.1 S1.1 U4.2
GND2 [power]: C7.2 C8.2 C9.2 D5.C D6.C J7.GND J7.GND2 J8.6 J9.10 Q5.2 R19.1 R20.1 R22.1 R24.1 S3.1 U6.2
GND3 [power]: C10.2 C11.2 C12.2 D7.C D8.C J10.GND J10.GND2 J11.6 J12.10 Q7.2 R28.1 R29.1 R31.1 R33.1 S4.1 U8.2
GND4 [power]: C13.2 C14.2 C15.2 D9.C D10.C J13.GND J13.GND2 J14.6 J15.10 Q9.2 R37.1 R38.1 R40.1 R42.1 S5.1 U10.2
GND5 [power]: C16.2 C17.2 C18.2 D11.C D12.C J16.GND J16.GND2 J17.6 J18.10 Q11.2 R46.1 R47.1 R49.1 R51.1 S6.1 U12.2
GND6 [power]: C19.2 C20.2 C21.2 D13.C D14.C J19.GND J19.GND2 J20.6 J21.10 Q13.2 R55.1 R56.1 R58.1 R60.1 S7.1 U14.2
GND7 [power]: C22.2 C23.2 C24.2 D15.C D16.C J22.GND J22.GND2 J23.6 J24.10 Q15.2 R64.1 R65.1 R67.1 R69.1 S8.1 U16.2
N$1: BUZZ.2 R7.1
N$2: LS1.- Q1.3
N$3: BUZZ.1 LS1.+
N$4: Q2.2 R1.2
N$5: Q1.1 R8.2 R9.2
N$6: PWR.1 R4.1
N$7: Q2.1 R10.2 R11.2
N$8: D2.A PWR_LED.1
N$9: D1.A R4.2
N$10: LS2.- Q3.3
N$11: Q3.1 R13.2 R14.2
N$12: Q4.2 R18.2
N$13: Q4.1 R15.2 R16.2
N$14: D4.A PWR_LED1.1
N$15: BUZZ1.2 R12.1
N$16: BUZZ1.1 LS2.+
N$17: PWR1.1 R17.1
N$18: D3.A R17.2
N$19: LS3.- Q5.3
N$20: Q5.1 R22.2 R23.2
N$21: Q6.2 R27.2
N$22: Q6.1 R24.2 R25.2
N$23: D6.A PWR_LED2.1
N$24: BUZZ2.2 R21.1
N$25: BUZZ2.1 LS3.+
N$26: PWR2.1 R26.1
N$27: D5.A R26.2
N$28: LS4.- Q7.3
N$29: Q7.1 R31.2 R32.2
N$30: Q8.2 R36.2
N$31: Q8.1 R33.2 R34.2
N$32: D8.A PWR_LED3.1
N$33: BUZZ3.2 R30.1
N$34: BUZZ3.1 LS4.+
N$35: PWR3.1 R35.1
N$36: D7.A R35.2
N$37: LS5.- Q9.3
N$38: Q9.1 R40.2 R41.2
N$39: Q10.2 R45.2
N$40: Q10.1 R42.2 R43.2
N$41: D10.A PWR_LED4.1
N$42: BUZZ4.2 R39.1
N$43: BUZZ4.1 LS5.+
N$44: PWR4.1 R44.1
N$45: D9.A R44.2
N$46: LS6.- Q11.3
N$47: Q11.1 R49.2 R50.2
N$48: Q12.2 R54.2
N$49: Q12.1 R51.2 R52.2
N$50: D12.A PWR_LED5.1
N$51: BUZZ5.2 R48.1
N$52: BUZZ5.1 LS6.+
N$53: PWR5.1 R53.1
N$54: D11.A R53.2
N$55: LS7.- Q13.3
N$56: Q13.1 R58.2 R59.2
N$57: Q14.2 R63.2
N$58: Q14.1 R60.2 R61.2
N$59: D14.A PWR_LED6.1
N$60: BUZZ6.2 R57.1
N$61: BUZZ6.1 LS7.+
N$62: PWR6.1 R62.1
N$63: D13.A R62.2
N$64: LS8.- Q15.3
N$65: Q15.1 R67.2 R68.2
N$66: Q16.2 R72.2
N$67: Q16.1 R69.2 R70.2
N$68: D16.A PWR_LED7.1
N$69: BUZZ7.2 R66.1
N$70: BUZZ7.1 LS8.+
N$71: PWR7.1 R71.1
N$72: D15.A R71.2
RXI: J3.9 J4.4
RXI1: J5.4 J6.9
RXI2: J8.4 J9.9
RXI3: J11.4 J12.9
RXI4: J14.4 J15.9
RXI5: J17.4 J18.9
RXI6: J20.4 J21.9
RXI7: J23.4 J24.9
STATUS_LED: J3.3 R11.1
STATUS_LED1: J6.3 R16.1
STATUS_LED2: J9.3 R25.1
STATUS_LED3: J12.3 R34.1
STATUS_LED4: J15.3 R43.1
STATUS_LED5: J18.3 R52.1
STATUS_LED6: J21.3 R61.1
STATUS_LED7: J24.3 R70.1
STATUS_OUT: J4.1 PWR_LED.2 R1.1
STATUS_OUT1: J5.1 PWR_LED1.2 R18.1
STATUS_OUT2: J8.1 PWR_LED2.2 R27.1
STATUS_OUT3: J11.1 PWR_LED3.2 R36.1
STATUS_OUT4: J14.1 PWR_LED4.2 R45.1
STATUS_OUT5: J17.1 PWR_LED5.2 R54.1
STATUS_OUT6: J20.1 PWR_LED6.2 R63.1
STATUS_OUT7: J23.1 PWR_LED7.2 R72.1
TXO: J3.8 J4.5
TXO1: J5.5 J6.8
TXO2: J8.5 J9.8
TXO3: J11.5 J12.8
TXO4: J14.5 J15.8
TXO5: J17.5 J18.8
TXO6: J20.5 J21.8
TXO7: J23.5 J24.8
USB_N: J2.A7 J2.B7 J3.7
USB_N1: J1.A7 J1.B7 J6.7
USB_N2: J7.A7 J7.B7 J9.7
USB_N3: J10.A7 J10.B7 J12.7
USB_N4: J13.A7 J13.B7 J15.7
USB_N5: J16.A7 J16.B7 J18.7
USB_N6: J19.A7 J19.B7 J21.7
USB_N7: J22.A7 J22.B7 J24.7
USB_P: J2.A6 J2.B6 J3.6
USB_P1: J1.A6 J1.B6 J6.6
USB_P2: J7.A6 J7.B6 J9.6
USB_P3: J10.A6 J10.B6 J12.6
USB_P4: J13.A6 J13.B6 J15.6
USB_P5: J16.A6 J16.B6 J18.6
USB_P6: J19.A6 J19.B6 J21.6
USB_P7: J22.A6 J22.B6 J24.6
